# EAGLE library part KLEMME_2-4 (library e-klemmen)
Klemme 2 4
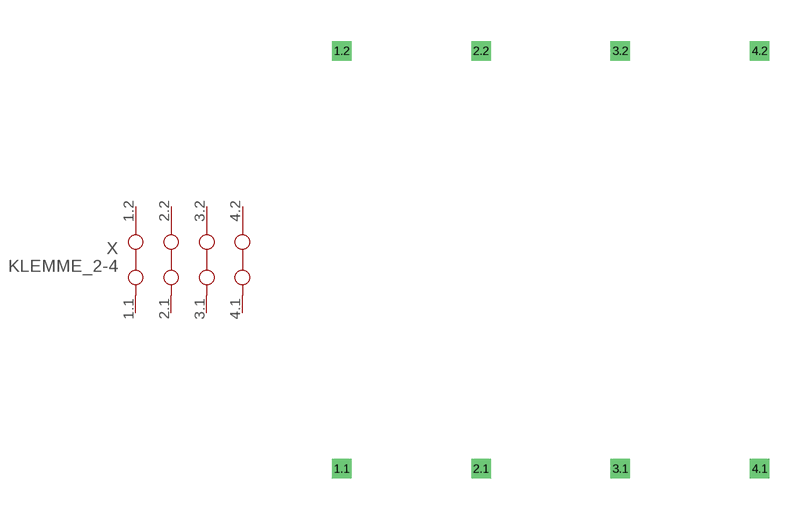
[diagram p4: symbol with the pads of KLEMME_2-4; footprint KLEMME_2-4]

Designator prefix X

## KLEMME_2-4  [KLEMME_2-4]
1.1  1.1  pas
1.2  1.2  pas
2.1  2.1  pas
2.2  2.2  pas
3.1  3.1  pas
3.2  3.2  pas
4.1  4.1  pas
4.2  4.2  pas

## Footprint KLEMME_2-4 (pad centres in mm)
Dummy
drill 0.2 pad 0.6 square: 1.1 0,-7.62; 1.2 0,7.62; 2.1 5.08,-7.62; 2.2 5.08,7.62; 3.1 10.16,-7.62; 3.2 10.16,7.62; 4.1 15.24,-7.62; 4.2 15.24,7.62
